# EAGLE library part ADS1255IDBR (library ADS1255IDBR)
24-Bit, 30kSPS, Very-Low-Noise Delta-Sigma ADC Source: Datasheet
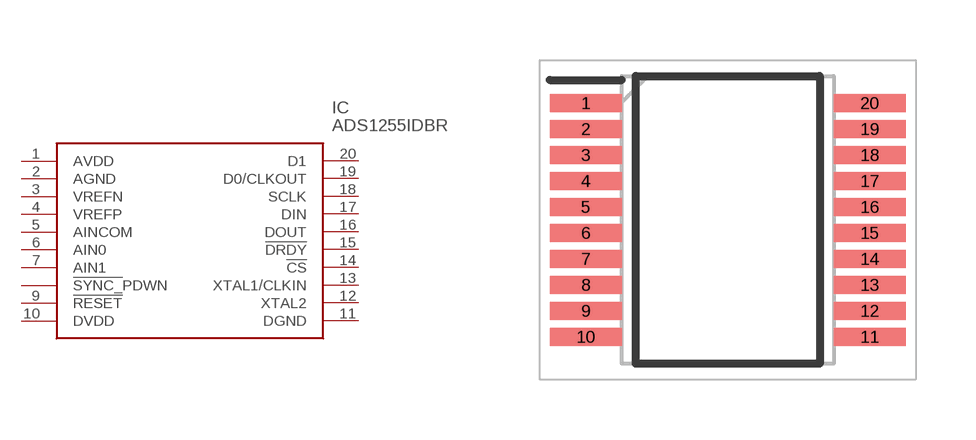
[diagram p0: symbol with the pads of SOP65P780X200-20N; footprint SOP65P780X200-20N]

Designator prefix IC

## ADS1255IDBR (Arrow_Part_Number: ADS1255IDBR; Arrow_Price-Stock: https://www.arrow.com/en/products/ads1255idbr/texas-instruments?region=nac; Description: 24-Bit, 30kSPS, Very-Low-Noise Delta-Sigma ADC; Height: 2mm; Manufacturer_Name: Texas Instruments; Manufacturer_Part_Number: ADS1255IDBR; Mouser_Part_Number: 595-ADS1255IDBR; Mouser_Price-Stock: https://www.mouser.co.uk/ProductDetail/Texas-Instruments/ADS1255IDBR?qs=RaXRGs7zCv5vXRtM5faqvA%3D%3D)  [SOP65P780X200-20N]
1  AVDD
2  AGND
3  VREFN
4  VREFP
5  AINCOM
6  AIN0
7  AIN1
8  !SYNC,_!PDWN  ?
9  !RESET
10  DVDD
11  DGND
12  XTAL2
13  XTAL1/CLKIN
14  !CS
15  !DRDY
16  DOUT
17  DIN
18  SCLK
19  D0/CLKOUT
20  D1

## Footprint SOP65P780X200-20N (pad centres in mm)
DB0020A
smd 1.8 x 0.45: 1 -3.55,2.925; 2 -3.55,2.275; 3 -3.55,1.625; 4 -3.55,0.975; 5 -3.55,0.325; 6 -3.55,-0.325; 7 -3.55,-0.975; 8 -3.55,-1.625; 9 -3.55,-2.275; 10 -3.55,-2.925; 11 3.55,-2.925; 12 3.55,-2.275; 13 3.55,-1.625; 14 3.55,-0.975; 15 3.55,-0.325; 16 3.55,0.325; 17 3.55,0.975; 18 3.55,1.625; 19 3.55,2.275; 20 3.55,2.925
